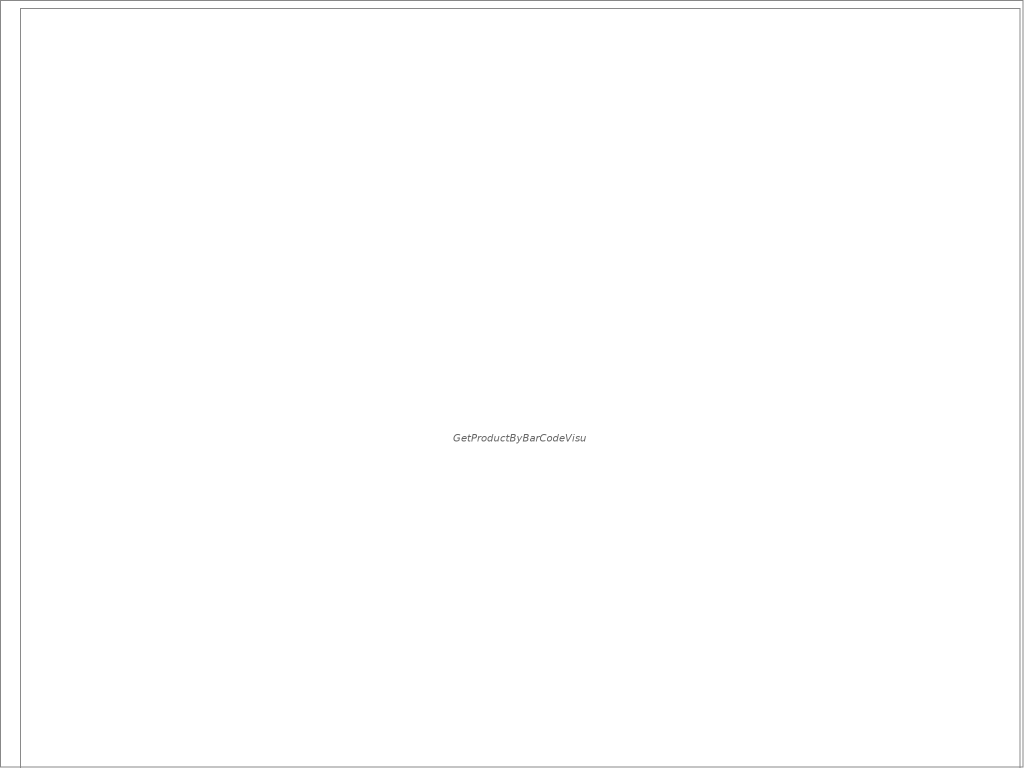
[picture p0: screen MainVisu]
VISUALIZATION MainVisu  // 1024x768
    TabControl (20,8 1000x860)
        shows GetProductByBarCodeVisu()
        shows GetPagedProductsVisu()
        shows AddProductVisu()
        shows DeleteProductVisu()
        shows UpdateProductVisu()
        [0]: TabTitle=根据BarCode获取产品
        [1]: TabTitle=查询分页数据
        [2]: TabTitle=添加产品
        [4]: TabTitle=根据条码更新产品数据
END_VISUALIZATION
